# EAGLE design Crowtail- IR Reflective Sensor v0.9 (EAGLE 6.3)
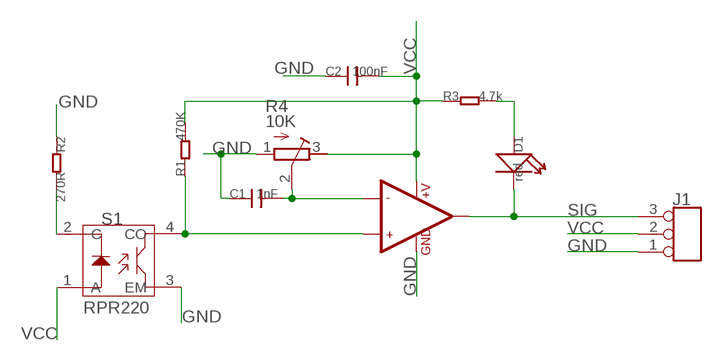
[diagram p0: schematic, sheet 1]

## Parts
C1  1nF  C-0603  [0603]
C2  100nF  C-0603  [0603]
D1  red  007-LED35*40  [LED0603]
J1  TINKER_3P_DIP  [3P_2.0_DIP]
R1  470K  005-R0603  [0603-1]
R2  270R  005-R0603_S  [0603_S]
R3  4.7k  005-R0603  [0603-1]
R4  10K  R-TRIMM3214W  [RTRIM3214W]
S1  RPR220  REFLECTIVE-PHOTOSENSOR-RPR-220  [4P-6.4X4.9X6.5H]
U1  002-LMV358  [SO08]

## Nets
GND: C1.1 C2.1 J1.1 R2.1 R4.1(E) S1.3(EM) U1.4(GND)
N$1: C1.2 R4.2(S) U1.2(-IN1)
N$2: R1.1 S1.4(CO) U1.3(+IN1)
N$5: R2.2 S1.2(C)
N$12: D1.1(+) R3.2
SIG: D1.2(-) J1.3 U1.1(OUT1)
VCC: C2.2 J1.2 R1.2 R3.1 R4.3(A) S1.1(A) U1.8(+V)
Unconnected: U1.5(+IN2) U1.6(-IN2) U1.7(OUT2)

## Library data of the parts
C1 C2 = Discrete:C*: Ceramic Capacitors
D1 = Discrete:007-LED*
J1 = Connector:TINKER_3P_DIP
R1-R3 = Discrete:005-R*
R4 = rcl:R-TRIMM: Trimm resistor
S1 = Discrete:REFLECTIVE-PHOTOSENSOR-RPR-220: http://wenku.baidu.com/view/18864e7d27284b73f24250aa.html
U1 = ICs:002-LMV358

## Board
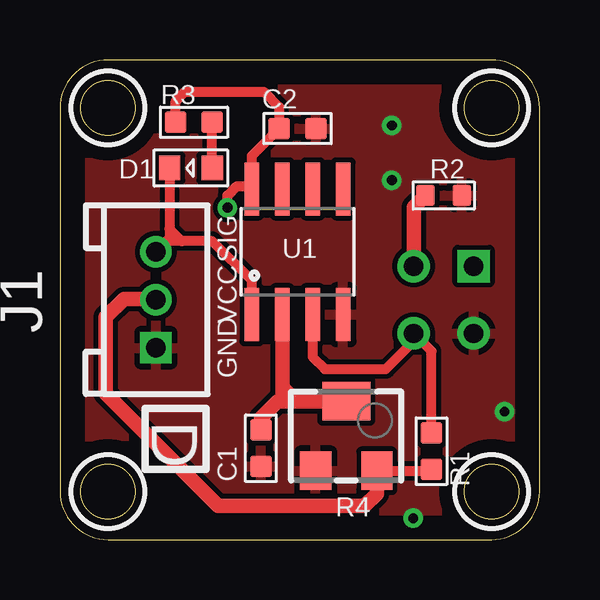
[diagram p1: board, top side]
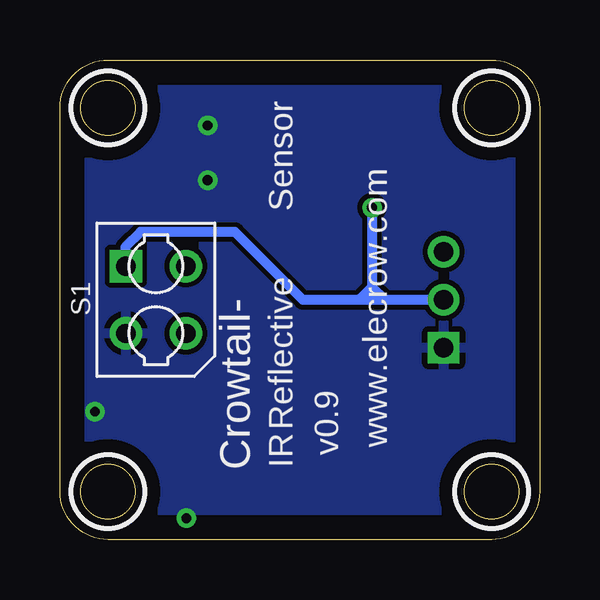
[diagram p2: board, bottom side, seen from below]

Size 20 x 20 mm. Coordinates in mm from the lower left corner, seen from the top.
Outline: 0,18 0,2 arc90 2,0 18,0 arc90 20,2 20,18 arc90 18,20 2,20 arc90 0,18
Outline: circle at 2,2 radius 1.14
Outline: circle at 18,2 radius 1.14
Outline: circle at 18,18 radius 1.14
Outline: circle at 2,18 radius 1.14
Copper layers (1*16): Top 0.035mm / dielectric 1.5mm / Bottom 0.035mm
Design rules "default *": minimum track width 10mil, minimum drill 24mil, track to track 8mil, track to pad 8mil, pad to pad 8mil, via to via 8mil, smd to smd 8mil, copper to edge 40mil, drill to drill 8mil, minimum pad ring 10mil, minimum via ring 8mil, stop-mask expansion 2mil, vias tented up to drill 100mil, thermal gap 10mil
tRestrict: area 0.5,0.5 to 3.5,3.5; area 16.5,0.5 to 19.5,3.5; area 16.5,16.5 to 19.5,19.5; area 0.5,16.5 to 3.5,19.5
bRestrict: area 0.5,0.5 to 3.5,3.5; area 16.5,0.5 to 19.5,3.5; area 16.5,16.5 to 19.5,19.5; area 0.5,16.5 to 3.5,19.5

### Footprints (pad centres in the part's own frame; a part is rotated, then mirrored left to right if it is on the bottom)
0603 = smd 0.889 x 0.889: 1 -0.762,0; 2 0.762,0
LED0603 = smd 0.889 x 1.016: 1 -0.889,0; 2 0.889,0
3P_2.0_DIP = drill 0.8 pad 1.27 square: 1 -2,0 | drill 0.8 pad 1.27: 2 0,0; 3 2,0
0603-1 = smd 0.889 x 0.889: 1 -0.762,0; 2 0.762,0
0603_S = smd 0.762 x 0.889: 1 -0.762,0; 2 0.762,0
RTRIM3214W = smd 1.3 x 1.6: 1 -1.275,-1.45; 3 1.275,-1.45 | smd 2 x 1.6: 2 0,1.45
4P-6.4X4.9X6.5H = drill 0.8 pad 1.35 square: 1 -1.4,-1.25 | drill 0.8 pad 1.35: 2 -1.4,1.25; 3 1.4,-1.25; 4 1.4,1.25
SO08 = smd 0.61 x 2.21: 1 -1.905,-2.616; 2 -0.635,-2.616; 3 0.635,-2.616; 4 1.905,-2.616; 5 1.905,2.616; 6 0.635,2.616; 7 -0.635,2.616; 8 -1.905,2.616

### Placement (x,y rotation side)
C1  8.38,3.81 90 top
C2  9.91,17.14 180 top
D1  5.46,15.49 180 top
J1  4,10 90 top
R1  15.49,3.68 270 top
R2  16,14.35 180 top
R3  5.59,17.4 0 top
R4  11.94,4.32 0 top
S1  16,10 270 bottom
U1  9.91,12 0 top

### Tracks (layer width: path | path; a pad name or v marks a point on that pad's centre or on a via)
GND  (via drill 0.41)
  other vias: 13.84,17.27 13.84,14.99 18.54,5.33 14.73,0.89
  pour Top: 0,0 20.32,0 20.32,20.32 0,20.32
  pour Bottom: 0,0 20.32,0 20.32,20.32 0,20.32
N$1
  Top 0.61: R4.2 9.27,5.77 | 9.27,5.77 9.07,5.77 8.38,5.08 C1.2 | U1.2 9.27,6.35 | 9.27,6.35 9.27,5.77 | 9.27,6.35 9.78,5.84
N$2
  Top 0.406: U1.3 10.54,7.62 11.05,7.11 13.59,7.11 14.75,8.27 S1.4 15.49,7.86 R1.1
N$5
  Top 0.61: S1.2 14.75,13.86 R2.2
N$12
  Top 0.406: D1.1 R3.2
SIG
  Top 0.406: D1.2 4.57,12.95 | 4.57,12.95 4.57,12.57 | 4.57,12.57 J1.3 4.45,12.45 5.08,12.45 | 4.57,12.57 3.94,11.94 | U1.1 8,10.79 6.35,12.45 5.08,12.45 | 4.57,12.95 5.08,12.45
VCC  (via drill 0.41)
  Top 0.406: R3.1 4.83,18.29 5.21,18.67 8.51,18.67 9.14,18.03 C2.2 8,16 U1.8 7.88,14.73 7.37,14.73 6.99,14.35 v6.99,13.84 | R4.3 15.44,2.87 R1.2
  Top 0.61: J1.2 3.97,10.03 2.67,10.03 1.91,9.27 1.91,6.1 6.6,1.4 12.7,1.4 13.21,1.91 R4.3
  Bottom 0.406: S1.1 17.27,11.42 17.27,12.19 16.64,12.83 12.7,12.83 9.87,10 6.99,10 | J1.2 6.99,10 | v6.99,13.84 6.99,10.54 | 6.99,10.54 6.99,10.41 | 6.99,10.41 6.99,10 | 6.99,10.41 7.37,10.03 | 6.99,10.54 6.48,10.03 | 6.99,10.54 7.49,10.03

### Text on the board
tPlace: SIG | VCC | GND | D
bPlace: Sensor | www.elecrow.com | v0.9 | Reflective | IR | Crowtail-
